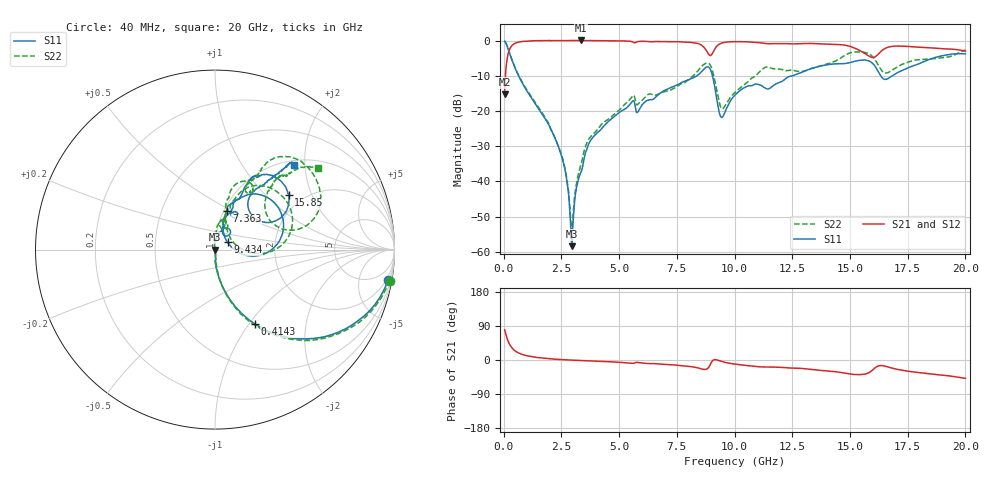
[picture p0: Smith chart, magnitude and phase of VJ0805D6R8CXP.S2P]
! VJ0805D6R8CXP
! DATE 10/29/2021  10:21
! CAPACITORS MOUNTED IN SERIES ON 25 MIL THICK MICROSTRIP SUBSTRATE
# GHz  S  MA  R  50.00
!  FREQ  S11M  S11A  S21M  S21A  S12M  S12A  S22M  S22A
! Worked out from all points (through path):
!   1601 points, 40 MHz to 20 GHz, reference 50 ohm
!   highest |S21| = 0.03 dB at 3.333 GHz (marker M1); lowest = -15.2 dB at 40 MHz (marker M2)
!   group delay of S21, straight-line fit = 7.4 ps
!   lowest |S11| = -58.4 dB at 2.959 GHz (marker M3), VSWR 1.00, Z = 50.1 + j0.0388 ohm
!   |S11| at or under -10 dB: 642.2 MHz to 8.368 GHz (7.726 GHz wide, 171 % of centre); 9.044 GHz to 12.51 GHz (3.469 GHz wide, 32.2 % of centre); 16.33 GHz to 16.83 GHz (509 MHz wide, 3.07 % of centre)
!   |S22| runs from -54.2 to -0.1 dB; largest |S21 - S12| = 0.0047
!   S11 on the Smith chart (normalised r, x): 40 MHz: 1, -11; 414.2 MHz: 1.00, -1.07; 7.363 GHz: 1.03, +0.46; 9.434 GHz: 1.15, +0.09; 15.85 GHz: 1.68, +1.38; 20 GHz: 1.08, +1.76
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0.04  0.9792 -9.9  0.1729 79.8  0.1736 80.1  0.9913 -10.1
0.202175  0.7423 -41.8  0.6666 48.1  0.6669 48.3  0.7512 -42.0
0.41425  0.4709 -61.7  0.8823 28.3  0.8812 28.3  0.4776 -62.1
2.36035  0.03158 -86.7  0.9985 1.6  0.9971 1.6  0.03185 -83.8
2.6847  0.01318 -87.1  0.9992 0.5  0.9978 0.5  0.01332 -78.4
2.95915  0.001203 18.8  0.9995 -0.3  0.9987 -0.3  0.001978 15.7
3.3334  0.01318 87.5  1.003 -1.4  1.002 -1.5  0.01678 93.0
3.370825  0.01419 90.2  1.002 -1.6  1.002 -1.6  0.01836 96.3
3.745075  0.03734 92.1  0.9983 -2.5  0.9974 -2.5  0.04216 88.3
4.493575  0.06889 83.8  0.9959 -4.4  0.9948 -4.4  0.07502 84.3
5.566425  0.136 63.4  0.9633 -8.8  0.9632 -8.8  0.1608 77.7
6.70165  0.1708 74.0  0.969 -10.4  0.968 -10.4  0.1737 73.3
7.362825  0.2234 73.3  0.9619 -13.0  0.9611 -13.0  0.209 72.5
8.8723  0.4194 27.6  0.644 -20.0  0.6426 -19.9  0.4768 27.7
9.433675  0.08103 30.5  0.9186 -3.7  0.9171 -3.6  0.1088 25.0
10.02  0.1676 72.3  0.9635 -11.0  0.9619 -11.0  0.1842 71.4
11.34235  0.2101 57.3  0.9085 -18.5  0.9086 -18.5  0.4175 66.1
13.35083  0.4038 63.9  0.9077 -25.1  0.9067 -25.1  0.4016 63.7
14.93515  0.481 59.0  0.8371 -36.2  0.8369 -36.4  0.6552 52.2
15.84582  0.5099 36.4  0.5953 -32.6  0.5937 -32.6  0.6413 23.8
16.68165  0.2927 50.1  0.8086 -19.0  0.8084 -19.2  0.3545 37.7
20  0.6467 47.1  0.7066 -48.2  0.7062 -48.3  0.7354 38.4
